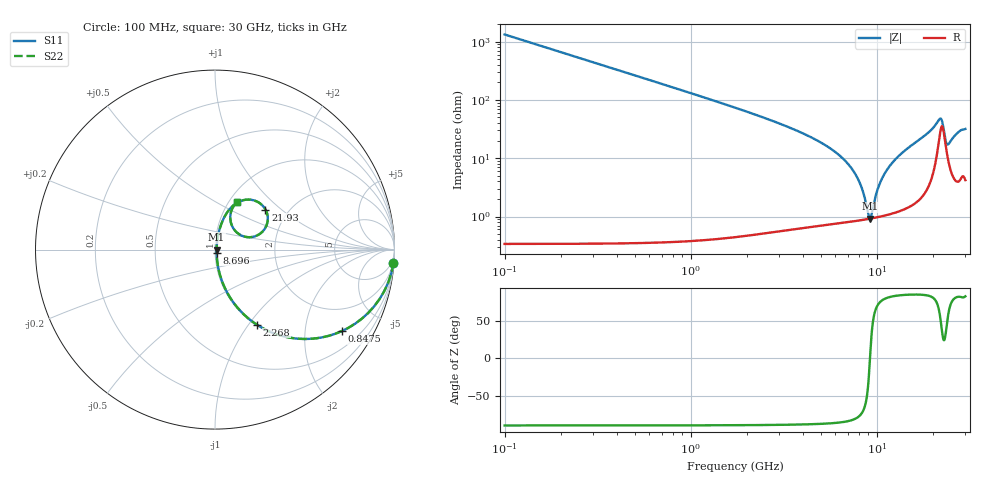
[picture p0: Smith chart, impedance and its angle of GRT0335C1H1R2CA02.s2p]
!Murata Part Number: GRT0335C1H1R2CA02
!These Parameters are Measured in Series Mode Connection
!Data Generated on Jun 19, 2026
!  o--ll--o
!Port1  Port2
!  o------o
!Operation Temp=25[degC], DC Bias Voltage=0[V]
!Freq. Start=100[MHz] Stop=30[GHz] 401[Steps]
# Hz S RI R 50
!Freq.(Hz) S11(Real) S11(Imag) S21(Real) S21(Imag) S12(Real) S12(Imag) S22(Real) S22(Imag)
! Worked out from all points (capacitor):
!   401 points, 100 MHz to 30 GHz, reference 50 ohm
!   read as one part in series: C = 1.2 pF near 249.5 MHz
!   lowest |Z| = 920 mohm at 9.22 GHz (marker M1)
!   series resonance near 9.211 GHz, so ESL is about 250 pH
!   S11 on the Smith chart (normalised r, x): 100 MHz: 1, -27; 847.5 MHz: 1.01, -3.10; 2.268 GHz: 1.01, -1.10; 8.696 GHz: 1.02, -0.03; 21.93 GHz: 1.54, +0.79; 30 GHz: 1.08, +0.63
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1e8  0.9943 -0.075  0.00567 0.075  0.00567 0.075  0.9943 -0.075
3.99e8  0.9165 -0.2762  0.0835 0.2762  0.0835 0.2762  0.9165 -0.2762
8.475e8  0.7059 -0.4544  0.2941 0.4544  0.2941 0.4544  0.7059 -0.4544
1.52025e9  0.4185 -0.4908  0.5815 0.4908  0.5815 0.4908  0.4185 -0.4908
2.26775e9  0.2331 -0.4184  0.7669 0.4184  0.7669 0.4184  0.2331 -0.4184
3.389e9  0.1064 -0.2998  0.8936 0.2998  0.8936 0.2998  0.1064 -0.2998
5.10825e9  0.0375 -0.1716  0.9625 0.1716  0.9625 0.1716  0.0375 -0.1716
7.4255e9  0.012 -0.0615  0.988 0.0615  0.988 0.0615  0.012 -0.0615
8.173e9  0.00972 -0.0341  0.9903 0.0341  0.9903 0.0341  0.00972 -0.0341
8.69625e9  0.0091 -0.0164  0.9909 0.0164  0.9909 0.0164  0.0091 -0.0164
9.2195e9  0.00911 0.000257  0.9909 -0.000257  0.9909 -0.000257  0.00911 0.000257
1.01165e10  0.0104 0.0269  0.9896 -0.0269  0.9896 -0.0269  0.0104 0.0269
1.0864e10  0.0124 0.0476  0.9876 -0.0476  0.9876 -0.0476  0.0124 0.0476
1.183575e10  0.0163 0.0729  0.9837 -0.0729  0.9837 -0.0729  0.0163 0.0729
1.505e10  0.0375 0.1487  0.9625 -0.1487  0.9625 -0.1487  0.0375 0.1487
2.005825e10  0.1325 0.2662  0.8675 -0.2662  0.8675 -0.2662  0.1325 0.2662
2.1927e10  0.281 0.2234  0.719 -0.2234  0.719 -0.2234  0.281 0.2234
2.289875e10  0.2334 0.0782  0.7666 -0.0782  0.7666 -0.0782  0.2334 0.0782
2.3721e10  0.1301 0.0886  0.8699 -0.0886  0.8699 -0.0886  0.1301 0.0886
2.50665e10  0.0861 0.1641  0.9139 -0.1641  0.9139 -0.1641  0.0861 0.1641
2.74585e10  0.1015 0.2387  0.8985 -0.2387  0.8985 -0.2387  0.1015 0.2387
3e10  0.1208 0.266  0.8792 -0.266  0.8792 -0.266  0.1208 0.266
